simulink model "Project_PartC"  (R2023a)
settings: Solver=FixedStepAuto  StartTime=0.0  StopTime=inf  FixedStep=.01  RelTol=1e-3  EnableMultiTasking=on
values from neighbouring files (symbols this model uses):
  encoderResolution = 48    [project_constants.m]
  gearRatio = 171.79    [project_constants.m]
  Kp = 250    [project_constants.m]
libraries: arduinolib x4, arduinosensorlib x1

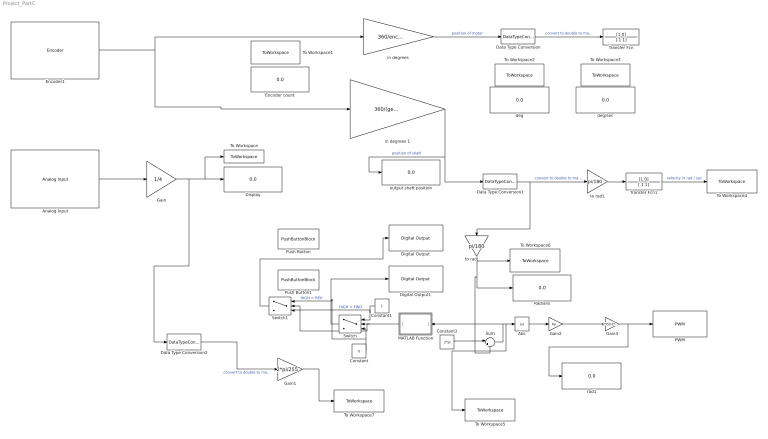
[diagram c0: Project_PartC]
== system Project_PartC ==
  Abs : Abs
  Analog Input : arduinolib/Analog Input  pinNumber=0  ReadResultsOnly=off  ConversionTriggerSource=Software  ExternalTriggerType=uint32( 0 )  OutputDataType=uint16  EnableConversionCompleteNotify=off  EnableOuputStatus=off  SampleTime=-1  blockPlatform=arduino
  Constant : Constant  Value=0
  Constant1 : Constant
  Constant2 : Constant  Value=2*pi
  Data Type Conversion : DataTypeConversion  OutDataTypeStr=double
  Data Type Conversion1 : DataTypeConversion  OutDataTypeStr=double
  Data Type Conversion2 : DataTypeConversion  OutDataTypeStr=double
  Digital Output : arduinolib/Digital Output  pinNumber=10  Direction=output  blockPlatform=arduino
  Digital Output1 : arduinolib/Digital Output  pinNumber=11  Direction=output  blockPlatform=arduino
  Display : Display
  Encoder count : Display
  Encoder1 : arduinosensorlib/Encoder  InputA=2  InputB=3  Mode=No reset  SampleTime=-1
  Gain : Gain  Gain=1/4
  Gain1 : Gain  Gain=2*pi/255
  Gain2 : Gain  Gain=Kp
  Gain3 : Gain  Gain=255/(2*pi)
  MATLAB Function : MATLAB Function  TreatAsAtomicUnit=on
  PWM : arduinolib/PWM  pinNumber=9  frequencyType=Default  desiredFrequency=490.2  achievableFrequency=490.2
  Push Button : PushButtonBlock  ButtonText=Pin2  OnValue=0  ButtonType=Latch  OffValue=1.000000
  Push Button1 : PushButtonBlock  ButtonText=Pin7  OnValue=0  ButtonType=Latch  OffValue=1.000000
  Radians : Display
  Sum : Sum  Inputs=|+-
  Switch : Switch  Criteria=u2 > Threshold
  Switch1 : Switch  Criteria=u2 > Threshold
  To Workspace : ToWorkspace  VariableName=pot_reading  SaveFormat=Structure With Time  SampleTime=-1
  To Workspace1 : ToWorkspace  VariableName=encoder_reading  SaveFormat=Structure With Time  SampleTime=-1
  To Workspace2 : ToWorkspace  VariableName=position  SaveFormat=Structure With Time  SampleTime=-1
  To Workspace3 : ToWorkspace  VariableName=speed  SaveFormat=Structure With Time  SampleTime=-1
  To Workspace4 : ToWorkspace  VariableName=shaft_speed  SaveFormat=Structure With Time  SampleTime=-1
  To Workspace5 : ToWorkspace  VariableName=error_signal  SaveFormat=Structure With Time  SampleTime=-1
  To Workspace6 : ToWorkspace  VariableName=shaft_position  SaveFormat=Structure With Time  SampleTime=-1
  To Workspace7 : ToWorkspace  VariableName=Theta_Des  SaveFormat=Structure With Time  SampleTime=-1
  Transfer Fcn : TransferFcn  Numerator=[1 0]  Denominator=[.1 1]
  Transfer Fcn1 : TransferFcn  Numerator=[1 0]  Denominator=[.1 1]
  deg : Display
  deg/sec : Display
  "in degrees " : Gain  Gain=360/encoderResolution
  in degrees 1 : Gain  Gain=360/(gearRatio*encoderResolution)
  output shaft position : Display
  rad1 : Display
  to rad : Gain  Gain=pi/180
  to rad1 : Gain  Gain=pi/180
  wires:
  Analog Input/1 -> Gain/1
  Gain/1 -> Data Type Conversion2/1, To Workspace/1, Display/1
  Encoder1/1 -> "in degrees "/1, in degrees 1/1
  Data Type Conversion/1 -> Transfer Fcn/1  "convert to double to make TF happy"
  "in degrees "/1 -> Data Type Conversion/1  "position of motor"
  in degrees 1/1 -> Data Type Conversion1/1, output shaft position/1  "position of shaft"
  Transfer Fcn1/1 -> To Workspace4/1  "velocity in rad / sec"
  Data Type Conversion1/1 -> to rad/1, to rad1/1  "convert to double to make TF happy"
  to rad/1 -> Sum/2, Radians/1, To Workspace6/1
  Gain1/1 -> To Workspace7/1
  Sum/1 -> To Workspace5/1, Abs/1, MATLAB Function/1(u)
  Data Type Conversion2/1 -> Gain1/1  "convert to double to make TF happy"
  Gain2/1 -> Gain3/1
  Gain3/1 -> rad1/1, PWM/1
  Abs/1 -> Gain2/1
  MATLAB Function/1(y) -> Switch1/2, Switch/2
  Constant1/1 -> Switch1/3, Switch/1  "HIGH = FWD"
  Switch/1 -> Digital Output1/1
  Constant/1 -> Switch1/1, Switch/3  "HIGH = REV"
  Switch1/1 -> Digital Output/1
  Constant2/1 -> Sum/1
  to rad1/1 -> Transfer Fcn1/1

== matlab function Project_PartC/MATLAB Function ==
function y = fcn(u)

y = u/abs(u);
